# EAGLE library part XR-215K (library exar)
Monolithic PHASE-LOCKED LOOP
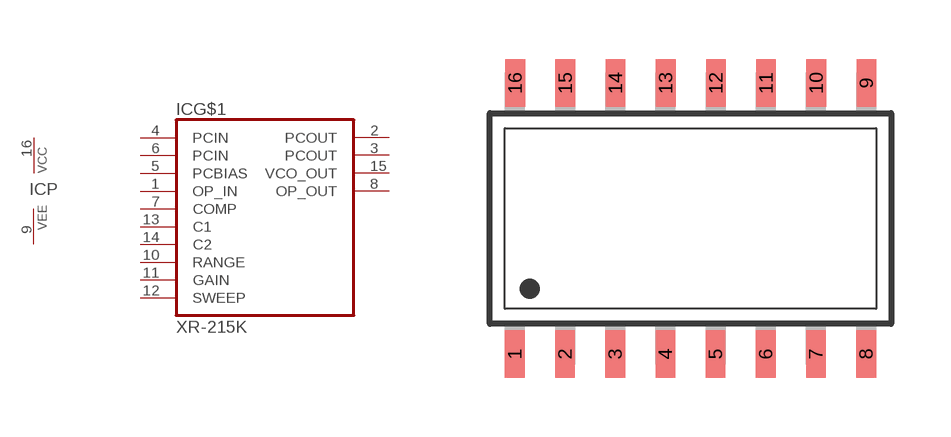
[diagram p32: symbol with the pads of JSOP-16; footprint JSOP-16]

Designator prefix IC; gates G$1=XR-215 P=PWR+/-

## XR-215K (OC_FARNELL: unknown; OC_NEWARK: unknown)  [JSOP-16]
1  G$1:OP_IN  in
2  G$1:PCOUT  out
3  G$1:PCOUT  out
4  G$1:PCIN  in
5  G$1:PCBIAS  in
6  G$1:PCIN  in
7  G$1:COMP  in
8  G$1:OP_OUT  out
9  P:VEE  pwr
10  G$1:RANGE  in
11  G$1:GAIN  in
12  G$1:SWEEP  in
13  G$1:C1  in
14  G$1:C2  in
15  G$1:VCO_OUT  out
16  P:VCC  pwr

## Footprint JSOP-16 (pad centres in mm)
JEDEC Small Outline Package
smd 0.5 x 1.2: 1 -4.445,-3.429; 2 -3.175,-3.429; 3 -1.905,-3.429; 4 -0.635,-3.429; 5 0.635,-3.429; 6 1.905,-3.429; 7 3.175,-3.429; 8 4.445,-3.429; 9 4.453,3.429; 10 3.183,3.429; 11 1.913,3.429; 12 0.643,3.429; 13 -0.627,3.429; 14 -1.897,3.429; 15 -3.167,3.429; 16 -4.437,3.429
